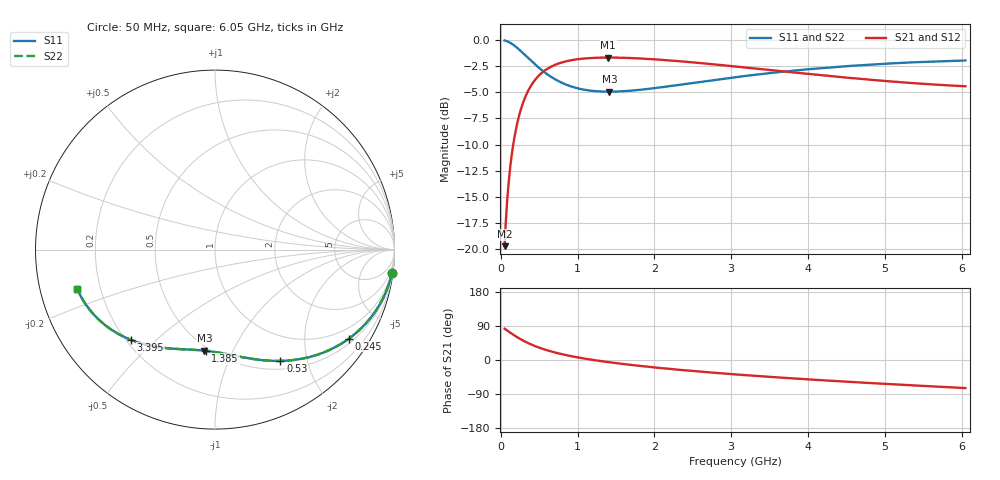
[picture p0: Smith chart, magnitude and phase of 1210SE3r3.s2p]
! AVX Thin Film Operation		Date: August 2001
! Description: Accu-P® Series, Thin Film, SMD, RF Capacitor
! Part Number: 12101J3R3ABT
! 50 MHz  -  6.05 GHz
! Serial Measurements
# mhz S db R 50
!	S11		S21		S12		S22
!	dB	Phase	dB	Phase	dB	Phase	dB	Phase
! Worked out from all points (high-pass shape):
!   401 points, 50 MHz to 6.05 GHz, reference 50 ohm
!   highest |S21| = -1.68 dB at 1.4 GHz (marker M1); lowest = -19.7 dB at 50 MHz (marker M2)
!   |S21| within 3 dB of the highest: 369.1 MHz to end of sweep
!   lowest |S11| = -4.9 dB at 1.415 GHz (marker M3), VSWR 3.61, Z = 23.6 - j39.1 ohm
!   |S11| at or under -10 dB: nowhere
!   |S22| runs from -4.9 to 0.0 dB; largest |S21 - S12| = 0
!   S11 on the Smith chart (normalised r, x): 50 MHz: 1, -15; 245 MHz: 0.64, -3.20; 530 MHz: 0.61, -1.57; 1.385 GHz: 0.48, -0.79; 3.395 GHz: 0.22, -0.42; 6.05 GHz: 0.11, -0.14
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50  -0.05 -7.4  -19.70 82.6  -19.70 82.6  -0.05 -7.4
110  -0.22 -16.1  -13.07 73.9  -13.07 73.9  -0.22 -16.1
140  -0.35 -20.2  -11.14 69.8  -11.14 69.8  -0.35 -20.2
185  -0.58 -26.2  -9.02 63.8  -9.02 63.8  -0.58 -26.2
245  -0.95 -33.6  -7.06 56.4  -7.06 56.4  -0.95 -33.6
365  -1.78 -46.2  -4.74 43.8  -4.74 43.8  -1.78 -46.2
530  -2.86 -59.5  -3.17 30.5  -3.17 30.5  -2.86 -59.5
635  -3.43 -66.2  -2.63 23.8  -2.63 23.8  -3.43 -66.2
755  -3.95 -72.6  -2.24 17.3  -2.24 17.3  -3.95 -72.6
890  -4.37 -78.7  -1.98 11.3  -1.98 11.3  -4.37 -78.7
1055  -4.71 -85.0  -1.79 5.0  -1.79 5.0  -4.71 -85.0
1385  -4.94 -95.2  -1.68 -5.2  -1.68 -5.2  -4.94 -95.2
1400  -4.94 -95.6  -1.68 -5.6  -1.68 -5.6  -4.94 -95.6
1415  -4.94 -96.0  -1.68 -6.0  -1.68 -6.0  -4.94 -96.0
1715  -4.83 -103.4  -1.74 -13.4  -1.74 -13.4  -4.83 -103.4
2060  -4.55 -110.8  -1.88 -20.8  -1.88 -20.8  -4.55 -110.8
2540  -4.07 -119.7  -2.17 -29.7  -2.17 -29.7  -4.07 -119.7
3050  -3.56 -127.9  -2.53 -37.9  -2.53 -37.9  -3.56 -127.9
3395  -3.26 -133.0  -2.79 -43.0  -2.79 -43.0  -3.26 -133.0
4055  -2.77 -141.8  -3.28 -51.8  -3.28 -51.8  -2.77 -141.8
5060  -2.25 -153.5  -3.95 -63.6  -3.95 -63.6  -2.25 -153.5
6050  -1.96 -164.0  -4.42 -74.1  -4.42 -74.1  -1.96 -164.0
